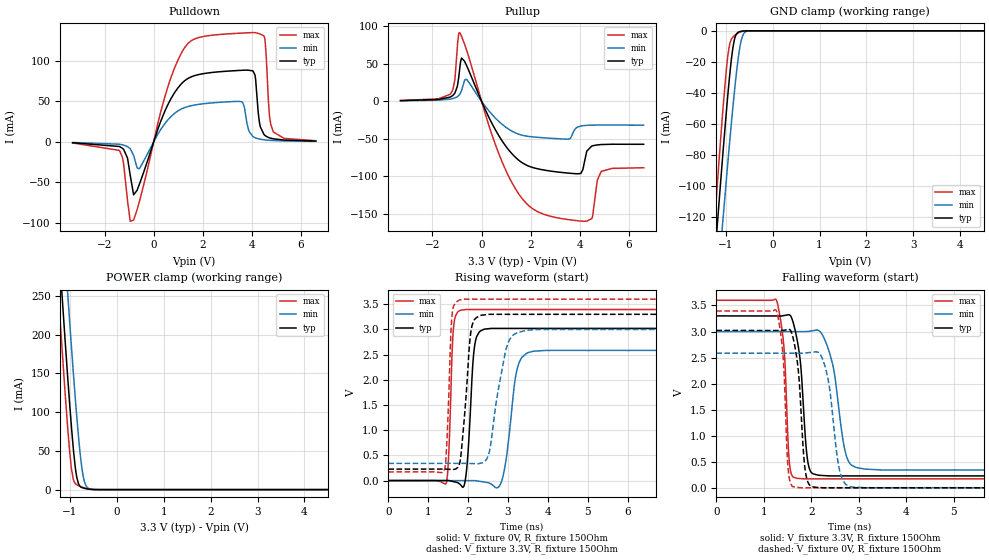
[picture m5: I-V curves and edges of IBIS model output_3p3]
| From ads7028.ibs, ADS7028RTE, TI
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|   output_3p3 Model
[Model]   output_3p3
Model_type   3-state
Polarity   Non-Inverting
Vmeas = 1.65
Vref = 0
Cref = 2pF
Rref = 100000
|   typ   min   max
C_comp   1.275pF   1.258pF   1.299pF
| Where Nom  PVT is Nominal Process, 3.3V, 27C
|   Fast PVT is Strong Process,  3.6V, -40C
|   Slow PVT is Weak Process,   3.0V, 125C
[Voltage Range]   3.3   3   3.6
|Junction Temperature
[Temperature Range]   27   125   -40
[Pullup Reference]   3.3   3   3.6
[Pulldown Reference]   0   0   0
[Power Clamp Reference]   3.3   3   3.6
[GND Clamp Reference]   0   0   0
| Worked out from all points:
|   slope of the pulldown table from 0 to 0.495 V, typ, clamps not added: 12.2 ohm
|   slope of the pullup table from 0 to 0.495 V, typ, clamps not added: 14.6 ohm
|   GND clamp passes 1 mA (typ) near -0.74 V on its own axis
|   POWER clamp passes 1 mA (typ) near -0.64 V on its own axis
|   falling waveform, V_fixture 3.3V, R_fixture 150Ohm: 20-80 % time 155ps typ, 254ps min, 112ps max; typ from 3.3 V to 0.227 V
|   rising waveform, V_fixture 0V, R_fixture 150Ohm: 20-80 % time 126ps typ, 223ps min, 85.7ps max; typ from 0 V to 3.02 V
|   rising waveform, V_fixture 3.3V, R_fixture 150Ohm: 20-80 % time 172ps typ, 321ps min, 94.6ps max; typ from 0.227 V to 3.3 V
|   falling waveform, V_fixture 0V, R_fixture 150Ohm: 20-80 % time 136ps typ, 202ps min, 104ps max; typ from 3.02 V to 0 V
[Pulldown]
|   Voltage   I(typ)   I(min)   I(max)
-3.3V     -1.068mA   -742.8uA   -1.333mA
-1.399V   -5.681mA   -2.899mA   -10.49mA
-953.7mV  -41.5mA    -8.439mA   -98.18mA
-815.1mV  -65.46mA   -16.69mA   -96.63mA
-597.3mV  -53.66mA   -33.32mA   -75.52mA
1.244V    75.15mA    42.19mA    115.7mA
3.6V      88.5mA     49.41mA    134.5mA
4.046V    87.62mA    6.61mA     135.1mA
4.521V    8.294mA    2.481mA    128mA
4.709V    5.1mA      1.975mA    34.86mA
4.867V    3.829mA    1.683mA    12.63mA
6.6V      1.007mA    637.5uA    1.435mA
[GND Clamp]
|   Voltage   I(typ)   I(min)   I(max)
-3.3V     -1.016A    -995.5mA   -1.059A
-1.32V    -182.1mA   -219.4mA   -160.1mA
-1.201V   -134.3mA   -174.7mA   -108.9mA
-1.181V   -126.5mA   -167.3mA   -100.5mA
-1.063V   -80.49mA   -123.7mA   -52.27mA
-953.7mV  -41.29mA   -85.03mA   -16.09mA
-844.8mV  -10.72mA   -48.87mA   -4.001mA
-795.3mV  -3.746mA   -33.98mA   -2.647mA
-716.1mV  -679.9uA   -14.21mA   -1.14mA
-627mV    -126.9uA   -2.506mA   -267.4uA
-478.5mV  -4.851uA   -43.73uA   -7.574uA
6.6V      0A         0A         0A
[Pullup]
|   Voltage   I(typ)   I(min)   I(max)
-3.3V     861.3uA    604.4uA    1.053mA
-1.27V    5.716mA    2.95mA     9.693mA
-1.092V   10.74mA    4.416mA    27.77mA
-894.3mV  42.32mA    9.151mA    91.61mA
-617.1mV  48.09mA    29.21mA    68.9mA
848.1mV   -53.42mA   -31.06mA   -81.72mA
2.095V    -88.44mA   -47.5mA    -143.6mA
4.036V    -96.24mA   -33mA      -159.7mA
4.283V    -66.49mA   -32.08mA   -159.7mA
4.511V    -59.44mA   -31.79mA   -154.5mA
4.867V    -57.7mA    -31.64mA   -93.71mA
6.6V      -57.35mA   -31.86mA   -88.6mA
[POWER Clamp]
|   Voltage   I(typ)   I(min)   I(max)
-3.3V     2.327A     2.43A      2.264A
-1.241V   319.5mA    430.1mA    250mA
-1.181V   265mA      375.4mA    195.7mA
-1.102V   194mA      303.6mA    126mA
-1.043V   142.8mA    250.8mA    77.41mA
-963.6mV  79.47mA    182.6mA    25.98mA
-914.1mV  45.53mA    141.8mA    10.95mA
-854.7mV  16.67mA    96.03mA    6.395mA
-735.9mV  2.499mA    24.96mA    3.157mA
-646.8mV  1.116mA    4.144mA    1.475mA
-478.5mV  88.54uA    150uA      82.93uA
6.6V      0A         0A         0A
[Ramp]
R_load = 150
|   typ   min   max
dV/dt_r   1.81253/1.26449e-10   1.55044/2.22647e-10   2.0369/8.56495e-11
dV/dt_f   1.84366/1.54471e-10   1.5954/2.52573e-10   2.05717/1.12295e-10
[Falling Waveform]
V_fixture = 3.3V
V_fixture_min = 3V
V_fixture_max = 3.6V
R_fixture = 150Ohm
C_fixture = 0F
|   Time   V(typ)   V(min)   V(max)
0s        3.3V       3V         3.6V
1.264ns   3.299V     2.999V     3.609V
1.429ns   3.307V     2.999V     2.656V
1.554ns   3.312V     2.999V     377.9mV
1.851ns   1.316V     2.998V     172.8mV
1.981ns   323.4mV    3.008V     172.8mV
2.353ns   230.3mV    2.684V     172.8mV
2.789ns   229.5mV    502.2mV    172.8mV
3.465ns   229.5mV    344.5mV    172.7mV
150ns     227.2mV    341mV      171.4mV
[Rising Waveform]
V_fixture = 0V
V_fixture_min = 0V
V_fixture_max = 0V
R_fixture = 150Ohm
C_fixture = 0F
|   Time   V(typ)   V(min)   V(max)
0s        -77.02nV   -316.4nV   -90.32nV
1.452ns   609.7uV    -527.1uV   -49.74mV
1.64ns    -22.44mV   -595.5uV   3.089V
1.949ns   124.1mV    -707.3uV   3.394V
2.166ns   2.694V     -786.2uV   3.394V
2.574ns   3.019V     -67.34mV   3.394V
2.872ns   3.019V     80.02mV    3.394V
3.293ns   3.019V     2.369V     3.394V
3.947ns   3.019V     2.583V     3.394V
150ns     3.021V     2.584V     3.395V
[Rising Waveform]
V_fixture = 3.3V
V_fixture_min = 3V
V_fixture_max = 3.6V
R_fixture = 150Ohm
C_fixture = 0F
|   Time   V(typ)   V(min)   V(max)
0s        227.2mV    341mV      171.4mV
1.395ns   228.6mV    341.6mV    192.4mV
1.603ns   220mV      341.7mV    3.331V
1.796ns   374.6mV    341.8mV    3.585V
1.911ns   1.31V      341.9mV    3.599V
2.166ns   3.201V     336.1mV    3.599V
2.527ns   3.299V     555mV      3.599V
3.027ns   3.299V     2.779V     3.599V
3.772ns   3.299V     2.998V     3.599V
150ns     3.3V       3V         3.6V
[Falling Waveform]
|Gnd
V_fixture = 0V
V_fixture_min = 0V
V_fixture_max = 0V
R_fixture = 150Ohm
C_fixture = 0F
|   Time   V(typ)   V(min)   V(max)
0s        3.021V     2.584V     3.395V
1.264ns   3.02V      2.584V     3.405V
1.407ns   3.023V     2.584V     2.524V
1.528ns   3.047V     2.583V     245.3mV
1.802ns   1.188V     2.583V     1.503mV
1.965ns   52.88mV    2.597V     1.502mV
2.317ns   1.894mV    2.243V     1.498mV
2.648ns   1.89mV     181mV      1.495mV
3.171ns   1.883mV    3.083mV    1.489mV
150ns     -76.92nV   -12.56nV   -33.21nV
